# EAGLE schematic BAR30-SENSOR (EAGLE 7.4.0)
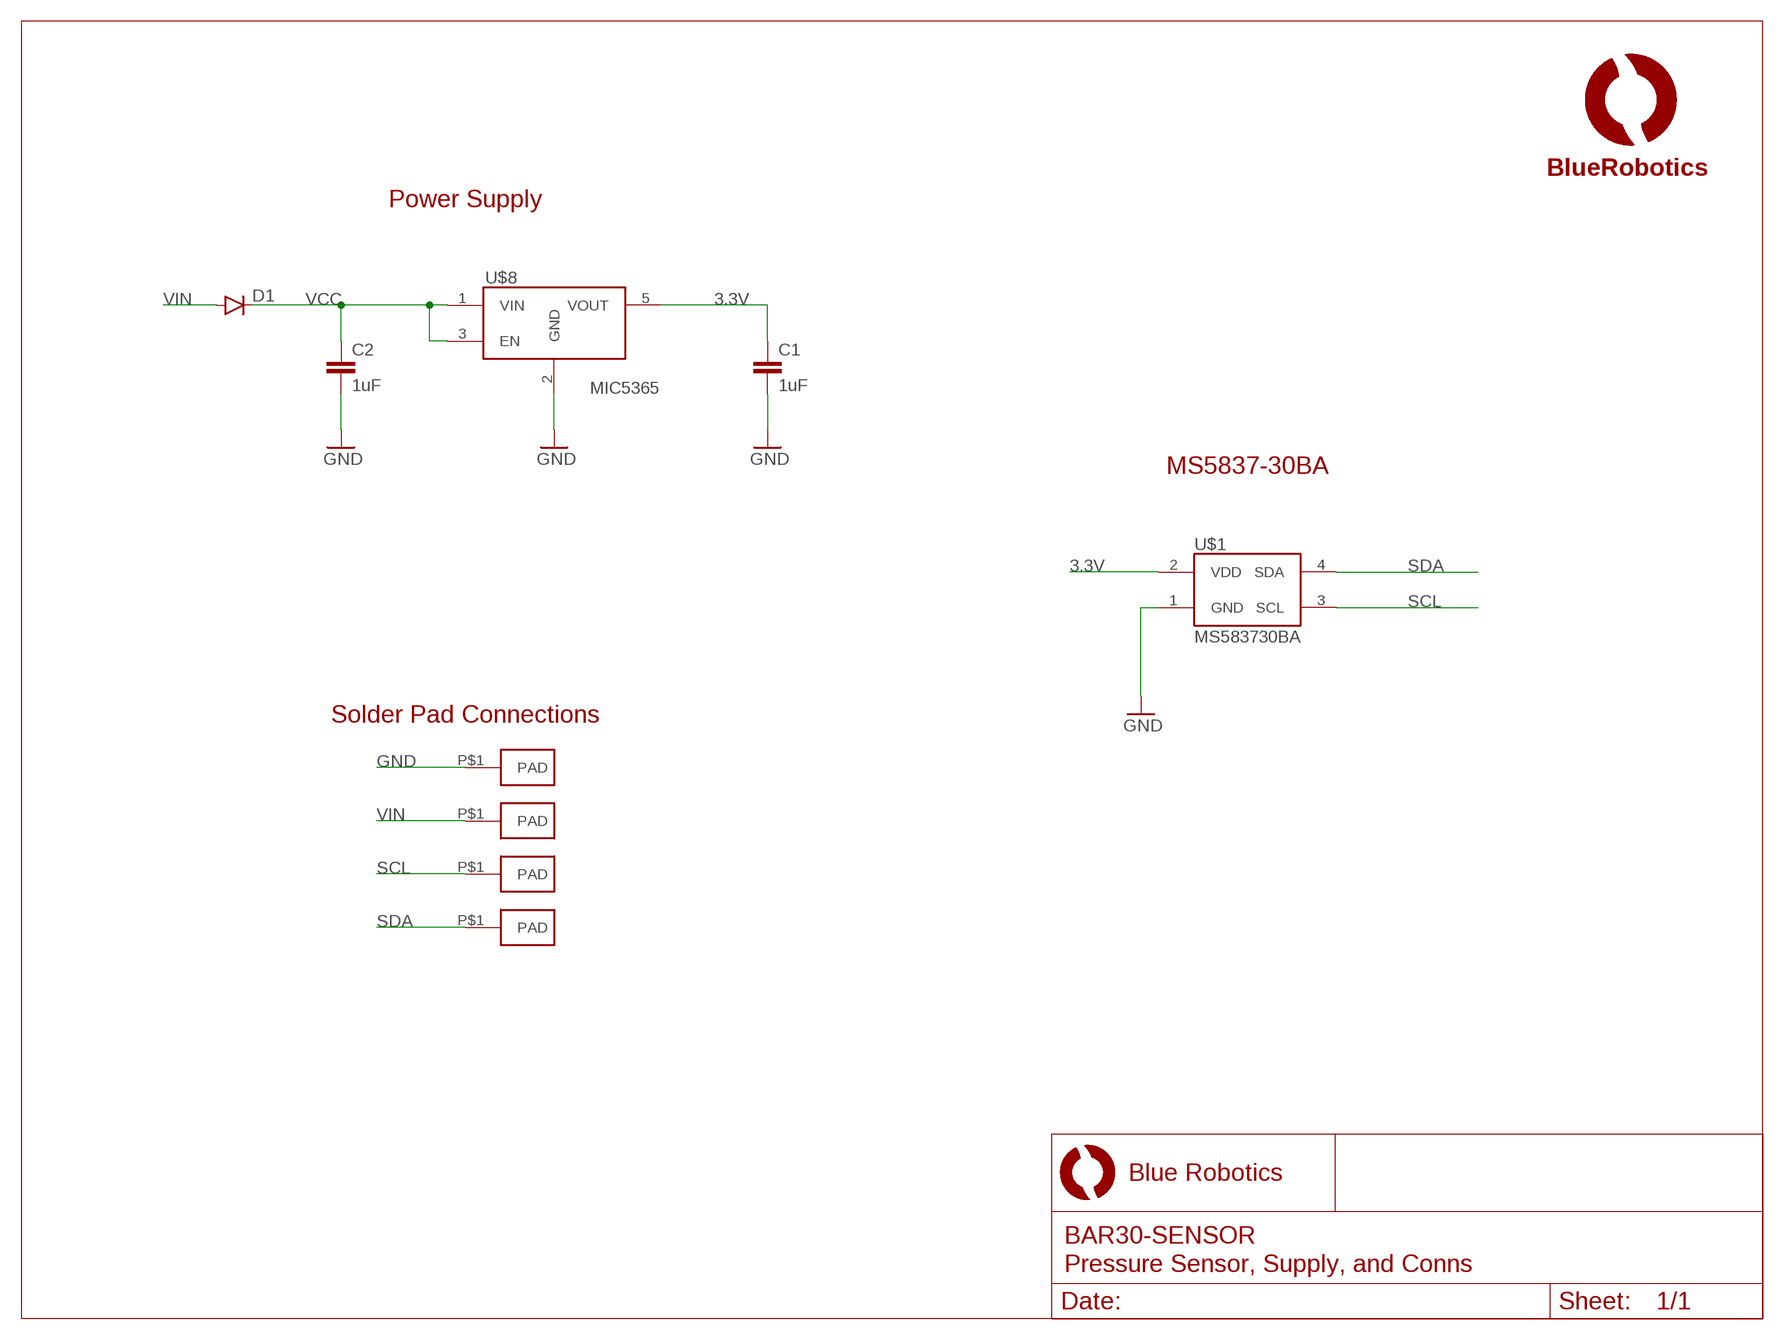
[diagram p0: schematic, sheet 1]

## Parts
C1  1uF  C-EUC0402  [C0402]
C2  1uF  C-EUC0402  [C0402]
D1  DIODESOD523  [SOD523]
U$1  MS583730BA  [MS5837]
U$3  PAD1.5X3MM  [PAD-1.5X3MM]
U$4  PAD1.5X3MM  [PAD-1.5X3MM]
U$5  PAD1.5X3MM  [PAD-1.5X3MM]
U$6  PAD1.5X3MM  [PAD-1.5X3MM]
U$7  LOGOBR-LOGO-S  [BR-LOGO-SMALL]
U$8  VREG-MIC5365  [SC70-5L]

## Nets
3.3V: C1.1 U$1.2(VDD) U$8.5(VOUT)
GND: C1.2 C2.2 U$1.1(GND) U$3.P$1(PAD) U$8.2(GND)
SCL: U$1.3(SCL) U$5.P$1(PAD)
SDA: U$1.4(SDA) U$6.P$1(PAD)
VCC: C2.1 D1.C U$8.1(VIN) U$8.3(EN)
VIN: D1.A U$4.P$1(PAD)

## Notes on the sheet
- Power Supply
- MIC5365
- MS5837-30BA
- Solder Pad Connections

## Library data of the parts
C1 C2 = resistor:C-EU: CAPACITOR, European symbol
D1 = SparkFun-DiscreteSemi:DIODE: Diode
U$1 = BR-Eagle-Library:MS5837
U$3-U$6 = BR-Eagle-Library:PAD
U$7 = BR-Eagle-Library:LOGO
U$8 = BlueRobotics-Main:VREG-MIC5365

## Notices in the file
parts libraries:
SparkFun-DiscreteSemi: Licensing: Creative Commons ShareAlike 4.0 International - https://creativecommons.org/licenses/by-sa/4.0
